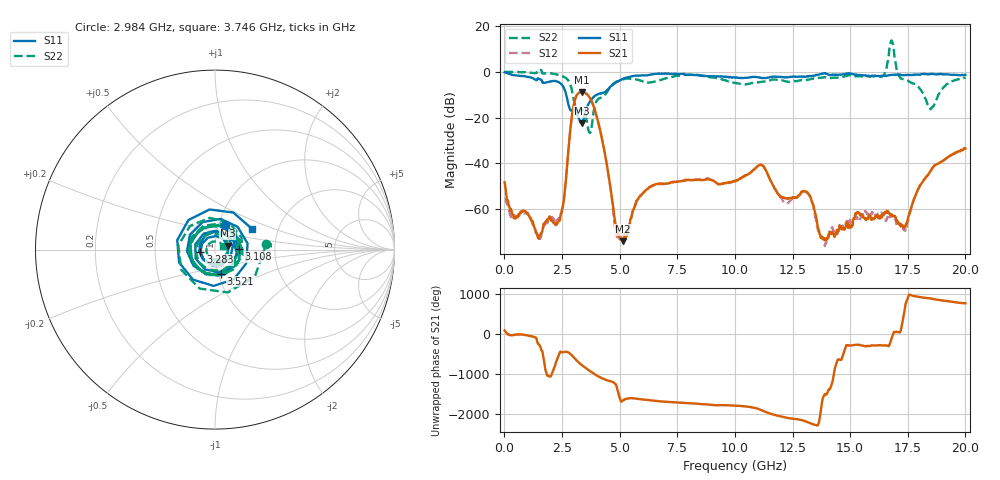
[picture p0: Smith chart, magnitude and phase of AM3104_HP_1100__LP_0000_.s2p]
!Created with skrf (http://scikit-rf.org).
# Hz S RI R 50.0
!freq ReS11 ImS11 ReS21 ImS21 ReS12 ImS12 ReS22 ImS22
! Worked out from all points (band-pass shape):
!   1601 points, 10 MHz to 20 GHz, reference 50 ohm
!   highest |S21| = -8.84 dB at 3.346 GHz (marker M1); lowest = -73.9 dB at 5.132 GHz (marker M2)
!   |S21| within 3 dB of the highest: 3.073 GHz to 3.736 GHz (663.1 MHz wide, 19.5 % of centre)
!   lowest |S11| = -22.6 dB at 3.346 GHz (marker M3), VSWR 1.16, Z = 57.6 + j2.59 ohm
!   |S11| at or under -10 dB: 2.68 GHz to 4.027 GHz (1.347 GHz wide, 40.2 % of centre)
!   |S22| runs from -26.7 to 13.6 dB; largest |S21 - S12| = 0.012
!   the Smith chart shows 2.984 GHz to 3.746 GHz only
!   S11 on the Smith chart (normalised r, x): 2.984 GHz: 1.08, +0.30; 3.108 GHz: 1.31, +0.01; 3.283 GHz: 0.85, -0.02; 3.521 GHz: 1.03, -0.28; 3.746 GHz: 1.46, +0.36
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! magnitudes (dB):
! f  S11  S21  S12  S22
! 10 MHz  -0.3  -48.2  -55.5  -0.1
! 1.459 GHz  -2.9  -72.4  -72.2  0.8
! 2.309 GHz  -4.4  -66.1  -64.8  -1.3
! 2.571 GHz  -6.9  -56.7  -56.1  -2.2
! 2.984 GHz  -16.7  -15.6  -15.7  -10.8
! 3.108 GHz  -17.5  -10.8  -10.8  -16.1
! 3.283 GHz  -21.7  -9.0  -9.1  -16.6
! 3.346 GHz  -22.6  -8.8  -8.9  -16.6
! 3.521 GHz  -17.2  -9.4  -9.4  -18.8
! 3.746 GHz  -12.6  -12.0  -12.1  -26.1
! 4.833 GHz  -4.8  -66.8  -69.6  -4.5
! 5.132 GHz  -3.2  -73.9  -70.8  -3.4
! 6.682 GHz  -0.9  -48.8  -49.0  -4.0
! 10.01 GHz  -2.6  -47.9  -47.5  -4.9
! 11.14 GHz  -2.7  -40.6  -40.8  -4.5
! 12.17 GHz  -2.5  -55.1  -57.1  -4.1
! 13.34 GHz  -1.9  -56.7  -56.7  -3.2
! 13.92 GHz  -0.6  -73.6  -74.9  -2.4
! 16.68 GHz  -1.5  -61.8  -64.4  7.1
! 17.38 GHz  -1.5  -67.7  -69.3  -3.6
! 18.48 GHz  -0.9  -43.5  -43.7  -16.2
! 20 GHz  -1.4  -33.5  -33.1  -2.7
